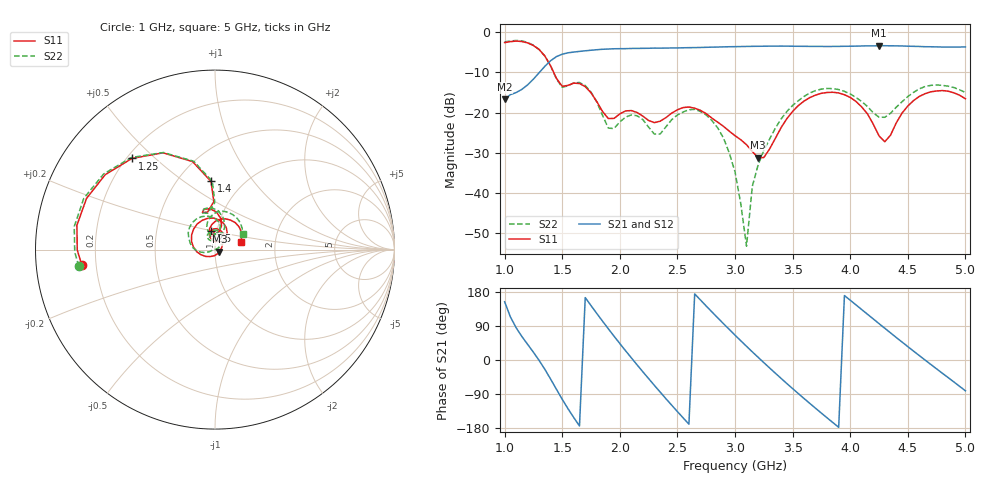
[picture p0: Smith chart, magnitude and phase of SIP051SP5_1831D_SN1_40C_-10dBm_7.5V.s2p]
# GHz  S  dB  R  50
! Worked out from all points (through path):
!   81 points, 1 GHz to 5 GHz, reference 50 ohm
!   highest |S21| = -3.31 dB at 4.25 GHz (marker M1); lowest = -16.7 dB at 1 GHz (marker M2)
!   lowest |S11| = -31.3 dB at 3.2 GHz (marker M3), VSWR 1.06, Z = 52.5 - j1.15 ohm
!   |S11| at or under -10 dB: 1.426 GHz to end of sweep
!   |S22| runs from -53.4 to -2.0 dB; largest |S21 - S12| = 0.0024
!   S11 on the Smith chart (normalised r, x): 1 GHz: 0.14, -0.05; 1.25 GHz: 0.22, +0.42; 1.4 GHz: 0.72, +0.64; 2.5 GHz: 0.93, +0.20; 5 GHz: 1.33, +0.12
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1  -2.53 -173.6  -16.72 153.8  -16.75 153.8  -2.33 -173.0
1.25  -3.26 132.3  -11.66 20.5  -11.66 20.5  -3.18 132.3
1.4  -8.38 93.4  -7.04 -50.7  -7.04 -50.8  -8.41 92.2
1.5  -13.45 101.3  -5.43 -103.7  -5.41 -103.6  -13.71 101.1
1.7  -13.53 88.0  -4.58 164.6  -4.58 164.5  -13.26 85.2
1.9  -21.50 89.0  -4.14 82.5  -4.13 82.5  -23.89 80.2
2.1  -19.51 99.2  -4.00 5.8  -4.00 5.6  -20.59 100.0
2.35  -22.18 106.9  -3.92 -84.5  -3.90 -84.6  -25.39 113.1
2.5  -19.33 102.7  -3.87 -136.1  -3.86 -136.0  -20.62 116.3
2.7  -19.46 68.9  -3.75 158.4  -3.75 158.3  -19.74 76.3
2.85  -22.42 49.4  -3.64 111.2  -3.65 111.2  -23.83 46.9
3  -25.80 35.8  -3.55 65.6  -3.53 65.7  -34.78 26.1
3.1  -28.05 17.7  -3.49 36.1  -3.50 36.1  -53.40 174.3
3.15  -29.72 1.8  -3.47 21.6  -3.47 21.7  -38.49 -171.5
3.2  -31.29 -23.7  -3.45 7.3  -3.45 7.3  -33.16 -163.5
3.45  -21.55 -160.2  -3.42 -62.1  -3.42 -62.0  -19.75 -177.0
3.7  -15.64 136.1  -3.49 -127.5  -3.49 -127.6  -14.52 139.3
3.95  -15.56 81.8  -3.45 170.0  -3.46 170.0  -14.72 96.2
4.25  -25.83 55.9  -3.31 96.0  -3.32 96.2  -21.16 88.0
4.35  -25.66 103.2  -3.33 71.7  -3.34 71.5  -20.20 107.5
4.65  -15.30 80.1  -3.56 -0.0  -3.55 -0.1  -13.51 86.3
5  -16.55 16.9  -3.61 -81.2  -3.61 -81.2  -15.00 30.2
